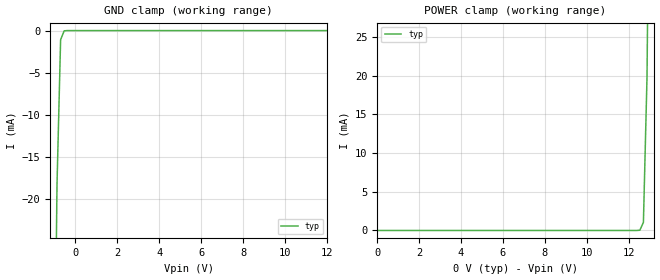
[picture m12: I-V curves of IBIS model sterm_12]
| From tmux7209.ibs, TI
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| sterm_12
[Model]   sterm_12
Model_type   Terminator
|   typ   min   max
C_comp   1.008417e-11   NA   NA
[Voltage Range]   12   0   12
[Temperature Range]   27   NA   NA
[Power Clamp Reference]   0   NA   NA
[GND Clamp Reference]   0   NA   NA
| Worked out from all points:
|   GND clamp passes 1 mA (typ) near -0.69 V on its own axis
[GND Clamp]
|   Voltage   I(typ)   I(min)   I(max)
-5V       -1.585A    NA         NA
-1.051V   -56.48mA   NA         NA
-878.8mV  -18.27mA   NA         NA
-707.1mV  -1.091mA   NA         NA
-535.4mV  -27.4uA    NA         NA
12V       293.5pA    NA         NA
[POWER Clamp]
|   Voltage   I(typ)   I(min)   I(max)
0V        -269.9pA   NA         NA
12.54V    32.05uA    NA         NA
12.71V    1.05mA     NA         NA
12.88V    19.88mA    NA         NA
13.05V    69.24mA    NA         NA
17V       3.279A     NA         NA
